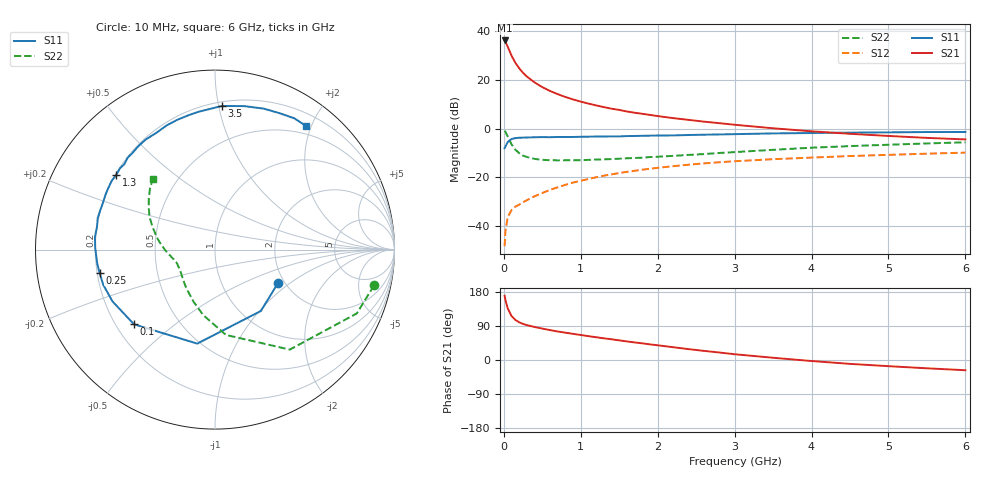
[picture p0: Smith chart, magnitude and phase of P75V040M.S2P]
! SIEMENS Small Signal Semiconductors
! BFP196
! Si NPN RF Bipolar Junction Transistor in SOT143
! VCE = 5 V  IC = 40 mA
! Common Emitter S-Parameters:  May  1996
# GHz  S  MA  R  50
!  f  S11  S21  S12  S22
! GHz  MAG  ANG  MAG  ANG  MAG  ANG  MAG  ANG
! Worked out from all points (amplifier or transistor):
!   36 points, 10 MHz to 6 GHz, reference 50 ohm
!   highest |S21| = 36.2 dB at 10 MHz (marker M1)
!   |S21| within 3 dB of that: start of sweep to 56.35 MHz
!   unconditionally stable (mu >= 1): 522.5 MHz to 4.205 GHz
!   at 250 MHz: K = 0.77, MSG = 26.5 dB, |S12| = -30.1 dB
!   at 1.4 GHz: K = 1.09, MAG = 11.7 dB, |S12| = -18.7 dB
!   at 6 GHz: K = 0.97, MSG = 2.7 dB, |S12| = -9.8 dB
!   S11 on the Smith chart (normalised r, x): 10 MHz: 1.85, -0.82; 100 MHz: 0.27, -0.37; 250 MHz: 0.21, -0.09; 1.3 GHz: 0.20, +0.32; 3.5 GHz: 0.23, +1.02; 6 GHz: 0.37, +1.92
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0.01  0.3975 -28.0  64.5 169.6  0.0039 80.3  0.9081 -12.7
0.02  0.427 -53.2  60.93 158.9  0.0078 72.3  0.8667 -24.2
0.05  0.5331 -100.7  48.21 136.4  0.0154 57.0  0.6958 -53.2
0.1  0.614 -137.3  31.45 116.1  0.0215 47.7  0.4792 -82.7
0.15  0.6399 -153.2  22.44 105.7  0.0253 46.7  0.3707 -100.2
0.2  0.6527 -162.5  17.31 99.4  0.0277 48.5  0.3146 -112.2
0.25  0.6562 -168.7  13.95 95.1  0.0311 49.8  0.2805 -121.7
0.3  0.6608 -173.3  11.71 92.0  0.0342 52.6  0.263 -128.4
0.4  0.6673 179.3  8.884 87.1  0.0412 56.2  0.2403 -138.7
0.5  0.6728 173.9  7.119 82.9  0.0479 58.2  0.23 -145.6
0.6  0.6696 169.1  5.939 78.9  0.0558 59.4  0.2258 -150.6
0.7  0.6767 164.9  5.119 75.2  0.0628 60.0  0.2244 -154.1
0.8  0.6758 160.9  4.473 72.1  0.0706 59.6  0.2249 -157.2
1.1  0.6864 150.1  3.272 62.9  0.0931 58.3  0.2293 -163.2
1.3  0.69 142.8  2.772 57.2  0.1089 56.4  0.2351 -166.5
1.7  0.7083 130.3  2.125 46.3  0.1371 51.7  0.2506 -172.4
2.2  0.7282 116.6  1.649 33.8  0.1703 44.9  0.2769 -179.1
2.8  0.7627 101.3  1.299 19.8  0.2051 36.4  0.3177 171.0
3.5  0.801 87.3  1.021 5.9  0.2369 26.8  0.369 160.3
4.5  0.8312 70.9  0.786 -10.2  0.2747 15.0  0.4396 147.2
5.5  0.8545 58.9  0.648 -21.9  0.3075 4.3  0.4989 136.4
6  0.8554 53.6  0.603 -27.0  0.323 -1.4  0.5256 131.1
